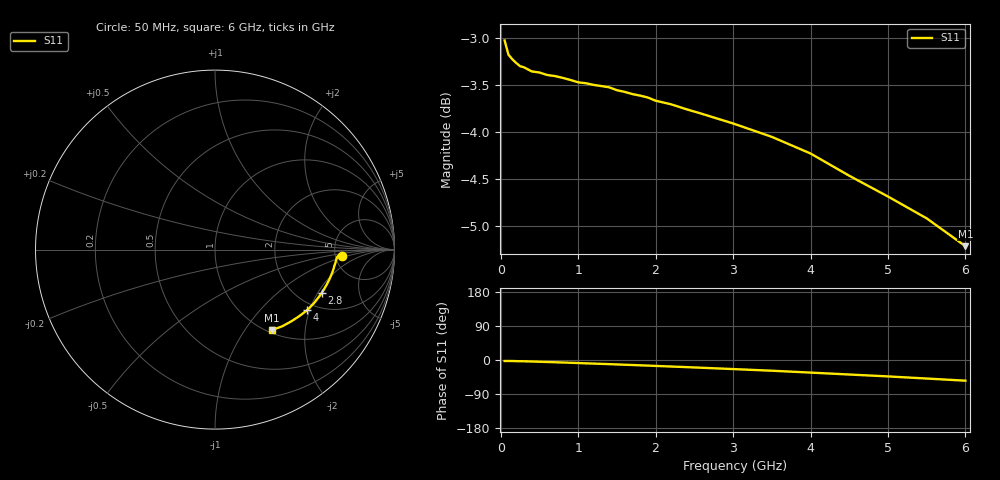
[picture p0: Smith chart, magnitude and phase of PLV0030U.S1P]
! Infineon Technologies  Discrete & RF Semiconductors
! BAR 64-04W /-05W /-06W
! Si PIN Diode in SOT323
! IF = 0.03 mA
! S-Parameters:  October  2008
# GHz  S  MA  R  50
!  f  S11
! GHz  MAG  ANG
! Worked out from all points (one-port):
!   34 points, 50 MHz to 6 GHz, reference 50 ohm
!   lowest |S11| = -5.2 dB at 6 GHz (marker M1), VSWR 3.43, Z = 52.5 - j67.3 ohm
!   |S11| at or under -10 dB: nowhere
!   S11 on the Smith chart (normalised r, x): 50 MHz: 5.69, -0.75; 2.8 GHz: 2.63, -2.17; 4 GHz: 1.78, -1.93; 6 GHz: 1.05, -1.35
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0.05  0.7057 -2.7
0.1  0.6934 -2.6
0.15  0.6896 -2.7
0.2  0.6865 -3.0
0.25  0.6838 -3.2
0.3  0.6829 -3.4
0.4  0.6795 -4.0
0.5  0.6786 -4.6
0.6  0.6765 -5.3
0.7  0.6757 -5.9
0.8  0.6742 -6.6
1  0.6705 -8.0
1.1  0.6698 -8.8
1.4  0.6664 -10.9
1.6  0.6627 -12.5
1.7  0.661 -13.2
1.9  0.6582 -14.8
2  0.6556 -15.6
2.2  0.6528 -17.2
2.4  0.6488 -18.8
2.8  0.6414 -22.2
3  0.6377 -23.9
3.5  0.6273 -28.3
4  0.6147 -33.2
4.5  0.5983 -38.3
5  0.5833 -43.3
5.5  0.5679 -48.9
6  0.549 -54.6
